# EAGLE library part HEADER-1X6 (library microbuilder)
PIN HEADER
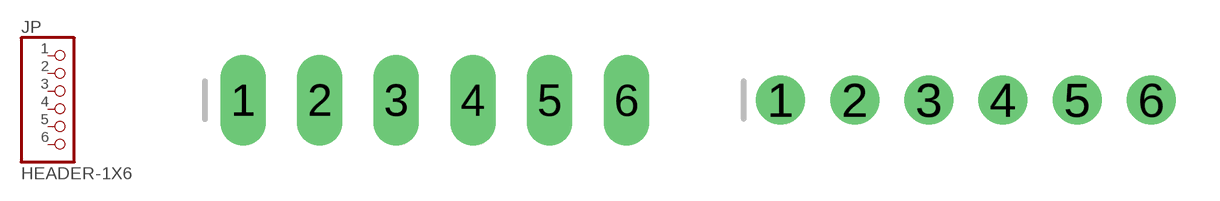
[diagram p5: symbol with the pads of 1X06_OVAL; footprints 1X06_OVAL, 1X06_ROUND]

Designator prefix JP

## HEADER-1X6  [1X06_OVAL]
1  1  pas
2  2  pas
3  3  pas
4  4  pas
5  5  pas
6  6  pas

## HEADER-1X6ROUND  [1X06_ROUND]
Pads as for 1X06_OVAL

## HEADER-1X6SMT  [1X06_SMT]
Pads as for 1X06_OVAL

## HEADER-1X676MIL  [1X06_ROUND_76]
Pads as for 1X06_OVAL

## HEADER-1X670MIL  [1X06_ROUND_70]
Pads as for 1X06_OVAL

## Footprint 1X06_OVAL (pad centres in mm)
PIN HEADER
drill 1 long: 1 -6.35,0; 2 -3.81,0; 3 -1.27,0; 4 1.27,0; 5 3.81,0; 6 6.35,0

## Footprint 1X06_ROUND (pad centres in mm)
PIN HEADER
drill 1 pad 1.676: 1 -6.35,0; 2 -3.81,0; 3 -1.27,0; 4 1.27,0; 5 3.81,0; 6 6.35,0

## Footprint 1X06_SMT (pad centres in mm)
Pin Headers 6 Pin, 0.1"/2.54mm pitch, SMT
smd 1 x 3.5: 1 -6.35,1.27; 2 -3.81,-1.27; 3 -1.27,1.27; 4 1.27,-1.27; 5 3.81,1.27; 6 6.35,-1.27

## Footprint 1X06_ROUND_76 (pad centres in mm)
drill 1 pad 1.93: 1 -6.35,0; 2 -3.81,0; 3 -1.27,0; 4 1.27,0; 5 3.81,0; 6 6.35,0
